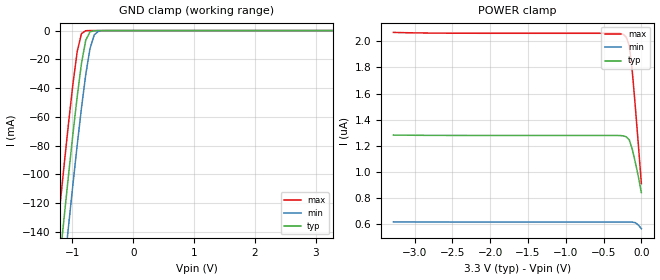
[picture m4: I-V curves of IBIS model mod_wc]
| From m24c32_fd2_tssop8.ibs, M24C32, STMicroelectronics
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|   Model mod_wc
[Model]   mod_wc
Model_type Input
Vinl   =   1.000V
Vinh   =   2.300V
C_comp   1.763pF   1.683pF   1.933pF
[Temperature Range]   25.0000   85.0000   -40.0000
[Voltage Range]   3.3000V   2.7000V   3.6000V
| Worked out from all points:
|   GND clamp passes 1 mA (typ) near -0.71 V on its own axis
[GND_clamp]
|Voltage   I(typ)   I(min)   I(max)
-3.3V     -1.086A    -1.119A    -1.052A
-1.27V    -186.8mA   -222.8mA   -150.3mA
-1.2V     -157.3mA   -193.3mA   -120.7mA
-1.13V    -128.1mA   -164mA     -91.65mA
-1.06V    -99.56mA   -135.2mA   -63.53mA
-920mV    -45.89mA   -79.74mA   -14.62mA
-850mV    -22.95mA   -53.94mA   -2.113mA
-780mV    -6.754mA   -30.77mA   -106.4uA
-710mV    -883.8uA   -12.62mA   -4.426uA
-640mV    -77.7uA    -2.974mA   -182.3nA
-570mV    -6.449uA   -439.9uA   -7.506nA
3.28V     6.813pA    40.1pA     6.666pA
[POWER_clamp]
|Voltage   I(typ)   I(min)   I(max)
-3.28V    1.283uA    617.8nA    2.068uA
-2.52V    1.28uA     616.7nA    2.062uA
-280mV    1.279uA    616.5nA    2.062uA
-240mV    1.277uA    616.5nA    2.053uA
-200mV    1.269uA    616.5nA    2.032uA
-160mV    1.246uA    616.5nA    1.967uA
-120mV    1.174uA    616.1nA    1.771uA
-80mV     1.073uA    612nA      1.501uA
-40mV     966.3nA    593.2nA    1.212uA
0V        842.2nA    566nA      911nA
